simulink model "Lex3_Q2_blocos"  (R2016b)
settings: Solver=ode45  StartTime=0.0  StopTime=Ts  RelTol=1e-6  EnableMultiTasking=on

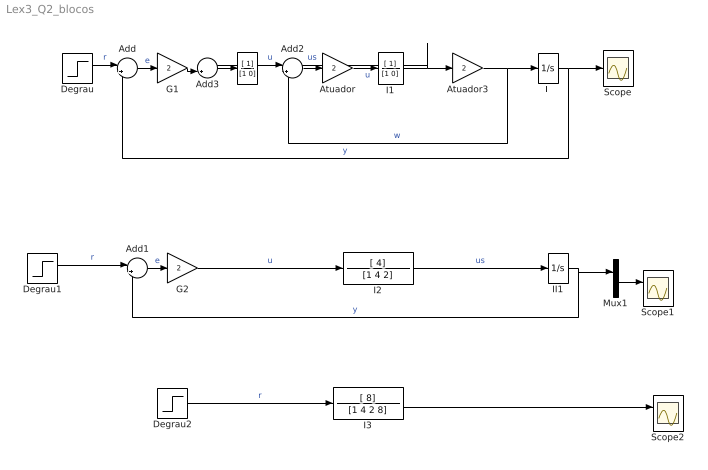
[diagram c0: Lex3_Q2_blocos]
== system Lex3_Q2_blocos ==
  Add : Sum  Inputs=|+-
  Add1 : Sum  Inputs=|+-
  Add2 : Sum  Inputs=|+-
  Add3 : Sum  Inputs=-+|
  Atuador : Gain  Gain=2
  Atuador3 : Gain  Gain=2
  Degrau : Step  After=2  SampleTime=0
  Degrau1 : Step  After=2  SampleTime=0
  Degrau2 : Step  After=2  SampleTime=0
  G1 : Gain  Gain=2
  G2 : Gain  Gain=2
  "I " : TransferFcn  Numerator=[ 1]  Denominator=[1 0]
  I1 : TransferFcn  Numerator=[ 1]  Denominator=[1 0]
  I2 : TransferFcn  Numerator=[ 4]  Denominator=[1 4 2]
  I3 : TransferFcn  Numerator=[ 8]  Denominator=[1 4 2 8]
  II : Integrator
  II1 : Integrator
  Mux1 : Mux  Inputs=2
  Scope : Scope
  Scope1 : Scope  NumInputPorts=2
  Scope2 : Scope  NumInputPorts=2
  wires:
  Add/1 -> G1/1  "e"
  Atuador3/1 -> Add2/2, II/1  "w"
  "I "/1 -> Add2/1  "u"
  Add2/1 -> Atuador/1
  Atuador/1 -> I1/1  "u"
  I1/1 -> Atuador3/1, Add3/1  "us"
  II/1 -> Scope/1, Add/2  "y"
  Degrau/1 -> Add/1  "r"
  G1/1 -> Add3/2
  Add3/1 -> "I "/1
  Add1/1 -> G2/1  "e"
  Mux1/1 -> Scope1/1
  I2/1 -> II1/1  "us"
  II1/1 -> Mux1/1, Add1/2  "y"
  Degrau1/1 -> Add1/1  "r"
  G2/1 -> I2/1  "u"
  I3/1 -> Scope2/1
  Degrau2/1 -> I3/1  "r"
